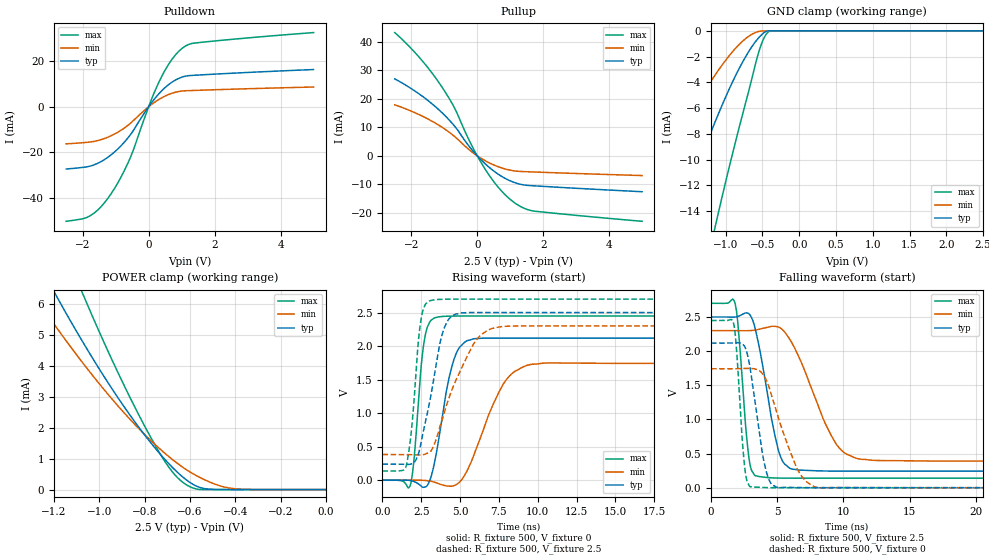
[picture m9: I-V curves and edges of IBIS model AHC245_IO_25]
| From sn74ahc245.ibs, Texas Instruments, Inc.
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[Model]   AHC245_IO_25
Model_type  I/O
Vinl = 0.5
Vinh = 1.7
Enable   Active-Low
|Vref =   0.0
|Rref =   1000
Cref =   50p
Vmeas =   1.25
| variable   typ   min   max
C_comp   2.58pF   2.42pF   2.69pF
| C_pullup   3.40pF   2.65pF   3.85pF
| C_pulldown   3.69pF   2.54pF   5.24pF
| C_tri-state   2.58pF   2.42pF   2.69pF
[Temperature Range]   40   100   -40
| Ambient temperature   25   85   -40
[Voltage range]   2.5   2.3   2.7
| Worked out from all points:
|   slope of the pulldown table from 0 to 0.375 V, typ, clamps not added: 56.2 ohm
|   slope of the pullup table from 0 to 0.375 V, typ, clamps not added: 89.9 ohm
|   GND clamp passes 1 mA (typ) near -0.62 V on its own axis
|   POWER clamp passes 1 mA (typ) near -0.71 V on its own axis
|   rising waveform, R_fixture 500, V_fixture 0: 20-80 % time 984ps typ, 1.84ns min, 518ps max; typ from 0.001 V to 2.12 V
|   falling waveform, R_fixture 500, V_fixture 2.5: 20-80 % time 1.26ns typ, 2.44ns min, 615ps max; typ from 2.5 V to 0.242 V
|   rising waveform, R_fixture 500, V_fixture 2.5: 20-80 % time 1.11ns typ, 1.95ns min, 541ps max; typ from 0.24 V to 2.5 V
|   falling waveform, R_fixture 500, V_fixture 0: 20-80 % time 957ps typ, 1.84ns min, 498ps max; typ from 2.12 V to 0.001 V
[GND Clamp]
| AHC245_IO_25
|   Voltage   I(typ)   I(min)   I(max)
-2.5V     -29.87mA   -17.99mA   -54.35mA
-2.25V    -25.3mA    -15.01mA   -46.62mA
-1.655V   -14.96mA   -8.352mA   -29.02mA
-1.14V    -7.027mA   -3.402mA   -15.15mA
-1.11V    -6.61mA    -3.152mA   -14.4mA
-870mV    -3.538mA   -1.387mA   -8.704mA
-630mV    -1.12mA    -224.6uA   -3.393mA
-560mV    -597uA     -61.78uA   -1.839mA
-505mV    -270.5uA   -13.94uA   -897.9uA
-450mV    -51.67uA   -8.977uA   -276.7uA
-395mV    -221.6nA   -5.293uA   -8.93uA
2.5V      40.87pA    60.87nA    34.5pA
[POWER Clamp]
| AHC245_IO_25
|   Voltage   I(typ)   I(min)   I(max)
-2.5V     28.07mA    22.13mA    38.78mA
-1.285V   7.55mA     6.242mA    10.21mA
-1.195V   6.33mA     5.298mA    8.509mA
-1.175V   6.066mA    5.094mA    8.141mA
-1.065V   4.673mA    4.017mA    6.189mA
-920mV    2.994mA    2.724mA    3.819mA
-790mV    1.673mA    1.709mA    1.919mA
-695mV    853.3uA    1.078mA    744.4uA
-635mV    428.6uA    740.4uA    257.4uA
-555mV    66.09uA    389.8uA    2.488uA
-430mV    794.3nA    55.84uA    120.5pA
-31.15fV  40.87pA    176pA      44.27pA
[Pulldown]
| AHC245_IO_25
|   Voltage   I(typ)   I(min)   I(max)
-2.5V     -27.28mA   -16.25mA   -50.19mA
-1.755V   -25.93mA   -15.41mA   -47.59mA
-1.45V    -24.09mA   -14.44mA   -43.88mA
-1.14V    -21.09mA   -12.71mA   -38.15mA
-850mV    -17.28mA   -10.42mA   -31.12mA
-570mV    -12.57mA   -7.447mA   -22.76mA
40mV      814uA      465.6uA    1.528mA
350mV     6.3mA      3.547mA    11.95mA
690mV     10.6mA     5.825mA    20.43mA
1.03V     13.07mA    6.925mA    25.76mA
1.365V    13.78mA    7.145mA    27.87mA
5V        16.31mA    8.66mA     32.51mA
[Pullup]
| AHC245_IO_25
|   Voltage   I(typ)   I(min)   I(max)
-2.5V     26.99mA    17.89mA    43.24mA
-1.795V   21.98mA    14.62mA    35.05mA
-1.18V    16.33mA    10.84mA    26.01mA
-925mV    13.48mA    8.894mA    21.54mA
-705mV    10.66mA    6.945mA    17.17mA
-210mV    2.829mA    1.793mA    4.636mA
200mV     -2.354mA   -1.442mA   -3.944mA
640mV     -6.489mA   -3.858mA   -11.07mA
1.08V     -9.17mA    -5.217mA   -16.05mA
1.395V    -10.19mA   -5.545mA   -18.28mA
1.71V     -10.53mA   -5.687mA   -19.4mA
5V        -12.61mA   -6.94mA    -22.99mA
[Ramp]
| AHC245_IO_25
| variable   typ   min   max
dV/dt_r   1.33/1.06E-09   1.10/1.98E-09   1.54/5.66E-10
dV/dt_f   1.39/1.33E-09   1.18/2.58E-09   1.57/6.46E-10
R_load = 500
[Rising Waveform]
| AHC245_IO_25
R_fixture =   500
C_fixture =   0
L_fixture =   0
V_fixture =   0
V_fixture_min = 0
V_fixture_max = 0
|   Time   V(typ)   V(min)   V(max)
0s        739.5uV    1.227mV    403.3uV
1.8ns     -3.776mV   1.274mV    -72.15mV
2.03ns    -17.78mV   1.705mV    298.9mV
2.69ns    -104.1mV   -1.628mV   2.068V
3.595ns   566.4mV    -48.07mV   2.434V
4.32ns    1.552V     -87.8mV    2.446V
5.01ns    1.993V     -17.7mV    2.448V
7.785ns   2.119V     1.435V     2.448V
9.555ns   2.118V     1.727V     2.448V
49.99ns   2.118V     1.741V     2.448V
[Falling Waveform]
| AHC245_IO_25
R_fixture =   500
C_fixture =   0
L_fixture =   0
V_fixture =   2.5
V_fixture_min = 2.3
V_fixture_max = 2.7
|   Time   V(typ)   V(min)   V(max)
0s        2.499V     2.299V     2.7V
1.815ns   2.498V     2.299V     2.701V
2.045ns   2.508V     2.299V     2.374V
2.83ns    2.552V     2.299V     493.9mV
3.385ns   2.292V     2.309V     172.3mV
5.115ns   530.7mV    2.35V      141.1mV
6.115ns   271.6mV    2.119V     139.9mV
9.265ns   243.1mV    701.1mV    139.9mV
11.16ns   242.2mV    421.8mV    139.9mV
49.99ns   242.3mV    389.2mV    140mV
[Rising Waveform]
| AHC245_IO_25
R_fixture =   500
C_fixture =   0
L_fixture =   0
V_fixture =   2.5
V_fixture_min = 2.3
V_fixture_max = 2.7
|   Time   V(typ)   V(min)   V(max)
0s        240.1mV    384.6mV    138.9mV
1.525ns   237.8mV    382.7mV    207.9mV
1.87ns    243.4mV    381.4mV    744.6mV
2.48ns    547.7mV    377.6mV    2.384V
3.19ns    1.351V     460.6mV    2.684V
3.77ns    2.107V     848.8mV    2.697V
4.31ns    2.411V     1.243V     2.699V
5.99ns    2.501V     2.072V     2.7V
7.55ns    2.5V       2.287V     2.7V
49.99ns   2.499V     2.299V     2.7V
[Falling Waveform]
| AHC245_IO_25
R_fixture =   500
C_fixture =   0
L_fixture =   0
V_fixture =   0
V_fixture_min = 0
V_fixture_max = 0
|   Time   V(typ)   V(min)   V(max)
0s        2.118V     1.741V     2.448V
1.72ns    2.119V     1.741V     2.397V
1.945ns   2.122V     1.742V     1.98V
2.525ns   2.072V     1.745V     339.4mV
2.985ns   1.717V     1.745V     12.91mV
4.08ns    313.4mV    1.612V     2.275mV
5.035ns   2.261mV    1.061V     91.42uV
6.615ns   2.001mV    238.9mV    -54.08uV
8.12ns    113.4uV    -970.9uV   -19.91uV
49.99ns   750.6uV    1.244mV    406.6uV
